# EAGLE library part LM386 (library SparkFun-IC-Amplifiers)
low voltage audio power amplifier SparkFun Products FabFM Radio Kit (KIT-11043)
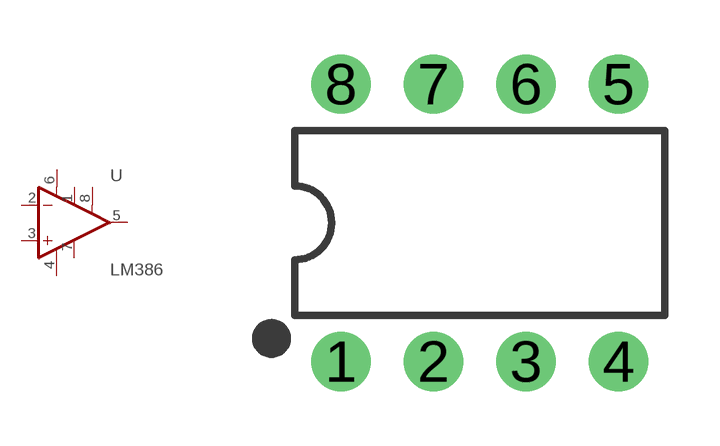
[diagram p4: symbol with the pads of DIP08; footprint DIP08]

Designator prefix U

## LM386 (PROD_ID: IC-10899; VALUE: LM386N)  [DIP08]
1  GAIN
2  -IN  in
3  +IN  in
4  V-  pwr
5  OUT  out
6  V+  pwr
7  BP
8  GAIN

## Footprint DIP08 (pad centres in mm)
Dual In Line Package
drill 0.813 pad 1.626: 1 -3.81,-3.81; 2 -1.27,-3.81; 3 1.27,-3.81; 4 3.81,-3.81; 5 3.81,3.81; 6 1.27,3.81; 7 -1.27,3.81; 8 -3.81,3.81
